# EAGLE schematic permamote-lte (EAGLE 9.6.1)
AUTHOR: NEAL JACKSON; REV: C; TITLE: PERMAMOTE

## Sheet 1 of 5: NRF
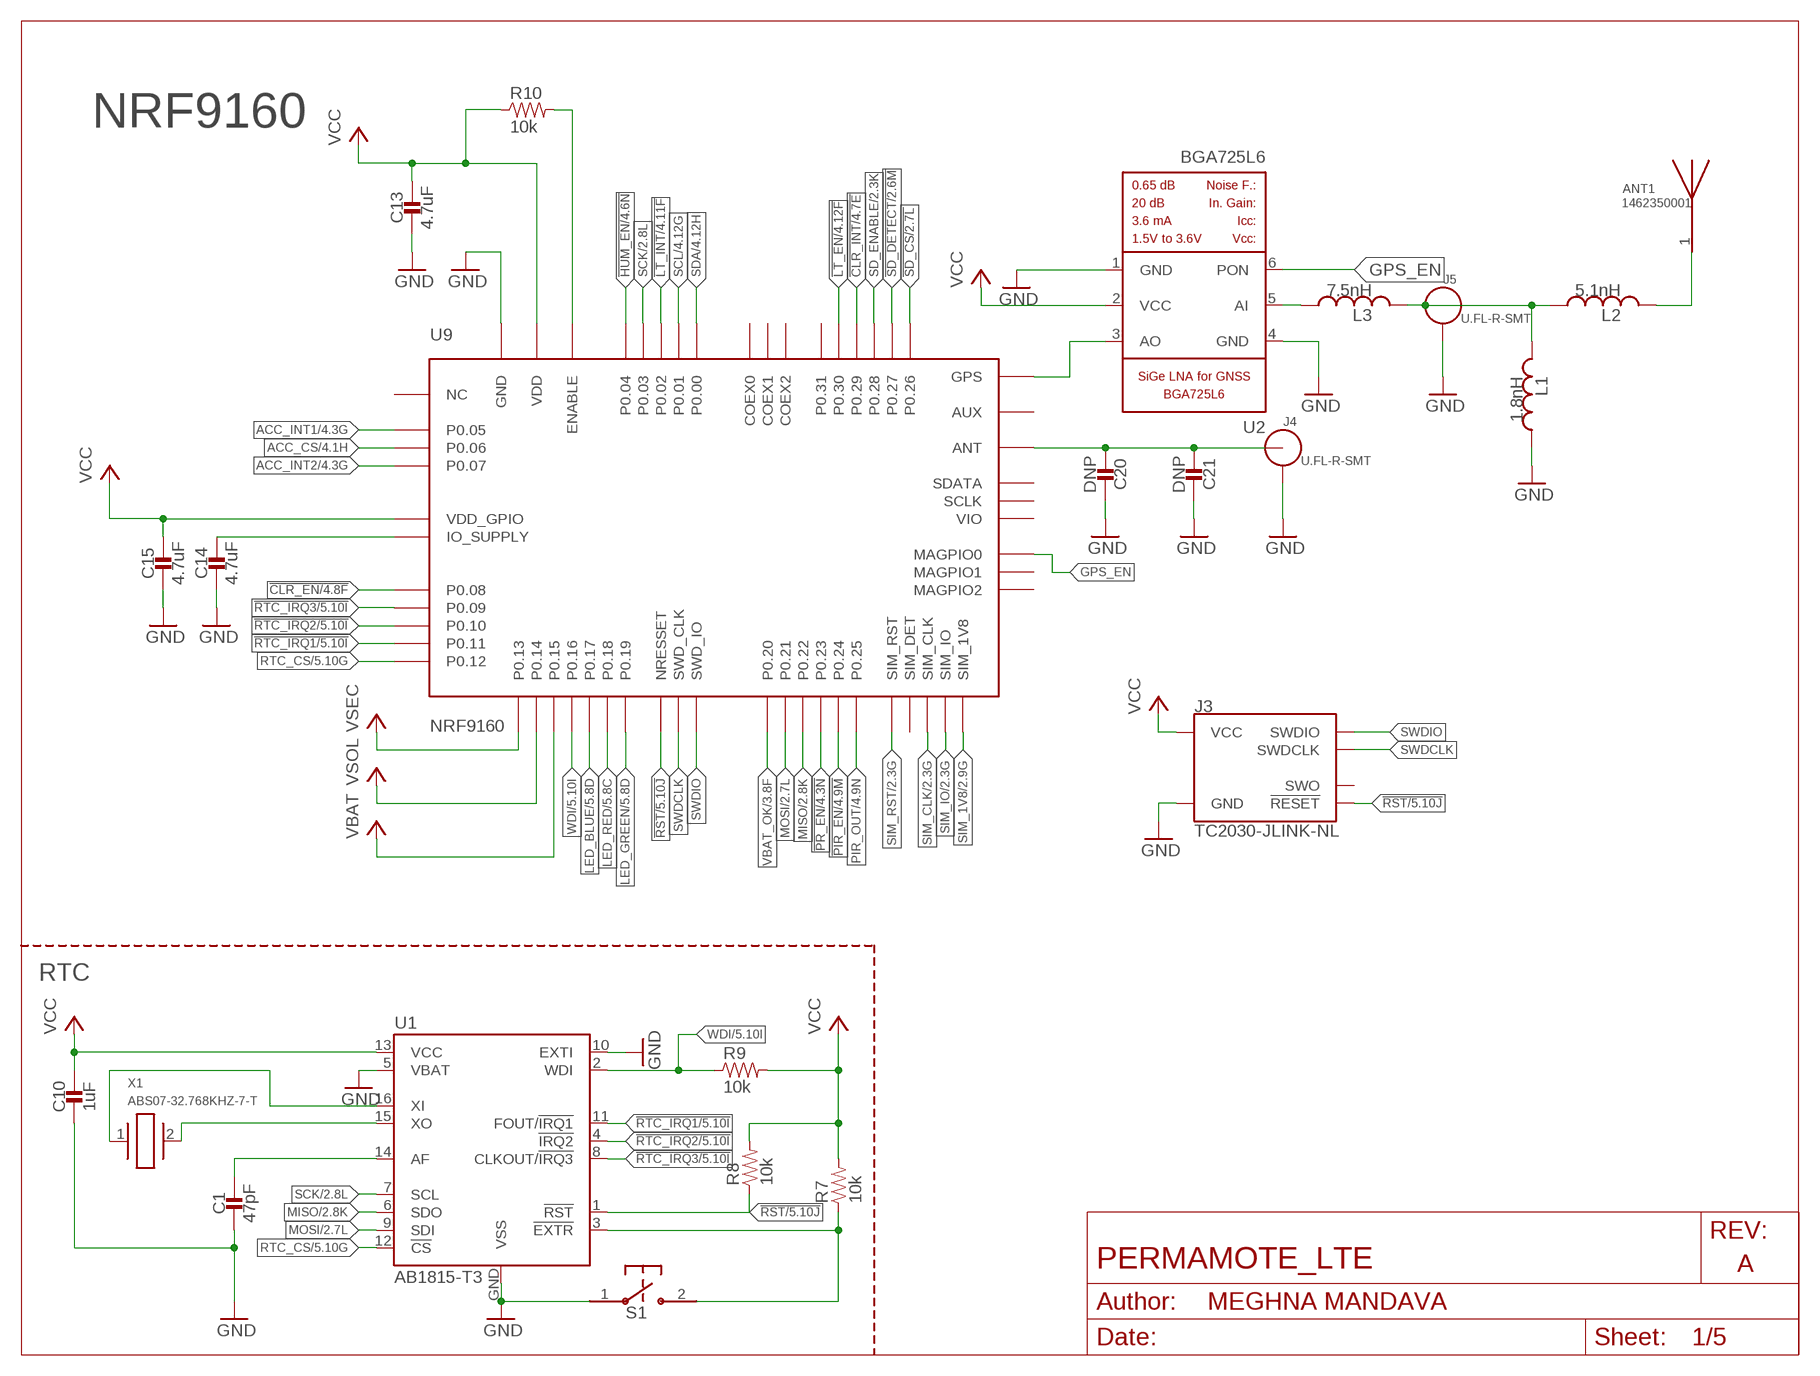
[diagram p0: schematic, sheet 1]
FRAME1 (LETTER_L_BLANK): AUTHOR: MEGHNA MANDAVA; REV: A; TITLE: PERMAMOTE_LTE

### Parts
ANT1  1462350001  [ANT_1462350001]
C1  47pF  CAPACITOR0402_CAP  [0402_CAP]
C10  1uF  CAPACITOR0402_CAP  [0402_CAP]
C13  4.7uF  CAPACITOR0402_CAP  [0402_CAP]
C14  4.7uF  CAPACITOR0402_CAP  [0402_CAP]
C15  4.7uF  CAPACITOR0402_CAP  [0402_CAP]
C20  DNP  CAPACITOR0402_CAP  [0402_CAP]
C21  DNP  CAPACITOR0402_CAP  [0402_CAP]
J3  TC2030-JLINK-NL  [TC2030-IDC-NL]
J4  U.FL-R-SMT  [U.FL_SMT]
J5  U.FL-R-SMT  [U.FL_SMT]
L1  1.8nH  INDUCTOR0402  [0402_CAP]
L2  5.1nH  INDUCTOR0402  [0402_CAP]
L3  7.5nH  INDUCTOR0402  [0402_CAP]
R7  10k  RESISTOR0402_RES  [0402_RES]
R8  10k  RESISTOR0402_RES  [0402_RES]
R9  10k  RESISTOR0402_RES  [0402_RES]
R10  10k  RESISTOR0402_RES  [0402_RES]
S1  B3U-1000P  [B3U-1000P]
U1  AB1815-T3  [QFN-16-3MM]
U2  BGA725L6  [LNA-TSLP-6-2-ORIG]
U9  NRF9160  [NRF9160]
X1  ABS07-32.768KHZ-7-T  [2-SMD]

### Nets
!CLR_EN: U9.P0.08 ; also sheet 4,5
!CLR_INT: U9.P0.29 ; also sheet 4,5
!HUM_EN: U9.P0.04 ; also sheet 4,5
!LT_EN: U9.P0.30 ; also sheet 4,5
!LT_INT: U9.P0.02 ; also sheet 4,5
!PIR_EN: U9.P0.24 ; also sheet 4,5
!PR_EN: U9.P0.23 ; also sheet 4,5
!RST: J3.3(!RESET) R8.1 U1.1(!RST) U9.NRESET(NRESSET) ; also sheet 5
!RTC_EXTR: R7.1 S1.2 U1.3(!EXTR)
!RTC_IRQ1: U1.11(FOUT/!IRQ1) U9.P0.11 ; also sheet 5
!RTC_IRQ2: U1.4(!IRQ2) U9.P0.10 ; also sheet 5
!RTC_IRQ3: U1.8(CLKOUT/!IRQ3) U9.P0.09 ; also sheet 5
!SD_CS: U9.P0.26 ; also sheet 2
!SD_DETECT: U9.P0.27 ; also sheet 2
ACC_CS: U9.P0.06 ; also sheet 4,5
ACC_INT1: U9.P0.05 ; also sheet 4,5
ACC_INT2: U9.P0.07 ; also sheet 4,5
GND: C1.2 C10.2 C13.2 C14.2 C15.2 C20.1 C21.1 J3.5(GND) J4.GND1 J4.GND2 J5.GND1 J5.GND2 L1.1 S1.1 U1.5(VBAT) U1.10(EXTI) U1.GND(VSS) U2.1(GND) U2.4(GND) U9.GND@1(GND) U9.GND@2(GND) U9.GND@3(GND) U9.GND@4(GND) U9.GND@5(GND) U9.GND@6(GND) U9.GND@7(GND) U9.GND@8(GND) U9.GND@9(GND) U9.GND@10(GND) U9.GND@11(GND) U9.GND@12(GND) U9.GND@13(GND) U9.GND@14(GND) U9.GND@15(GND) U9.GND@16(GND) U9.GND@17(GND) U9.GND@18(GND) U9.GND@19(GND) U9.GND@20(GND) U9.GND@21(GND) U9.GND@22(GND) U9.GND@23(GND) U9.GND@24(GND) U9.GND@25(GND) U9.GND@26(GND) U9.GND@27(GND) U9.GND@28(GND) U9.GND@29(GND) U9.GND@30(GND) U9.GND@31(GND) U9.GND@32(GND) U9.GND@33(GND) U9.GND@34(GND) U9.GND@35(GND) U9.GND_SHIELD@1(GND) U9.GND_SHIELD@2(GND) U9.GND_SHIELD@3(GND) U9.GND_SHIELD@4(GND) U9.GND_SHIELD@5(GND) U9.GND_SHIELD@6(GND) U9.GND_SHIELD@7(GND) U9.GND_SHIELD@8(GND) U9.GND_SHIELD@9(GND) U9.GND_SHIELD@10(GND) U9.GND_SHIELD@11(GND) U9.GND_SHIELD@12(GND) U9.GND_SHIELD@13(GND) U9.GND_SHIELD@14(GND) U9.GND_SHIELD@15(GND) U9.GND_SHIELD@16(GND) U9.GND_SHIELD@17(GND) U9.GND_SHIELD@18(GND) U9.GND_SHIELD@19(GND) U9.GND_SHIELD@20(GND) U9.GND_SHIELD@21(GND) U9.GND_SHIELD@22(GND) U9.GND_SHIELD@23(GND) U9.GND_SHIELD@24(GND) U9.GND_SHIELD@25(GND) U9.GND_SHIELD@26(GND) U9.GND_SHIELD@27(GND) U9.GND_SHIELD@28(GND) U9.GND_SHIELD@29(GND) U9.GND_SHIELD@30(GND) U9.GND_SHIELD@31(GND) U9.GND_SHIELD@32(GND) U9.GND_SHIELD@33(GND) U9.GND_SHIELD@34(GND) ; also sheet 2,3,4,5
GPS_EN: U2.6(PON) U9.MAGPIO0
LED_BLUE: U9.P0.17 ; also sheet 5
LED_GREEN: U9.P0.19 ; also sheet 5
LED_RED: U9.P0.18 ; also sheet 5
MISO: U1.6(SDO) U9.P0.22 ; also sheet 2,4,5
MOSI: U1.9(SDI) U9.P0.21 ; also sheet 2,4,5
N$1: U2.3(AO) U9.GPS
N$2: L3.1 U2.5(AI)
N$4: J5.SIG(ANT) L1.2 L2.1 L3.2
N$5: ANT1.1 L2.2
N$8: C20.2 C21.2 J4.SIG(ANT) U9.ANT
N$25: C1.1 U1.14(AF)
N$28: R10.2 U9.ENABLE
N$29: C14.1 U9.IO_SUPPLY
N$40: U1.15(XO) X1.2
N$43: U1.16(XI) X1.1
PIR_OUT: U9.P0.25 ; also sheet 4,5
RTC_CS: U1.12(!CS) U9.P0.12 ; also sheet 5
SCK: U1.7(SCL) U9.P0.03 ; also sheet 2,4,5
SCL: U9.P0.01 ; also sheet 4,5
SD_ENABLE: U9.P0.28 ; also sheet 2
SDA: U9.P0.00 ; also sheet 4,5
SIM_1V8: U9.SIM_1V8 ; also sheet 2
SIM_CLK: U9.SIM_CLK ; also sheet 2
SIM_IO: U9.SIM_IO ; also sheet 2
SIM_RST: U9.SIM_RST ; also sheet 2
SWDCLK: J3.4(SWDCLK) U9.SWDCLK(SWD_CLK)
SWDIO: J3.2(SWDIO) U9.SWDIO(SWD_IO)
VBAT: U9.P0.15 ; also sheet 3
VBAT_OK: U9.P0.20 ; also sheet 3
VCC: C10.1 C13.1 C15.1 J3.1(VCC) R7.2 R8.2 R9.2 R10.1 U1.13(VCC) U2.2(VCC) U9.VDD@1(VDD) U9.VDD@2(VDD) U9.VDD_GPIO ; also sheet 2,3,4,5
VSEC: U9.P0.13 ; also sheet 3
VSOL: U9.P0.14 ; also sheet 3,5
WDI: R9.1 U1.2(WDI) U9.P0.16 ; also sheet 5
Unconnected: J3.6(SWO) U9.AUX U9.COEX0 U9.COEX1 U9.COEX2 U9.MAGPIO1 U9.MAGPIO2 U9.NC1(NC) U9.NC2(NC) U9.NC3(NC) U9.NC4(NC) U9.NC5(NC) U9.NC6(NC) U9.NC7(NC) U9.NC8(NC) U9.NC9(NC) U9.NC10(NC) U9.NC11(NC) U9.NC12(NC) U9.NC13(NC) U9.NC14(NC) U9.NC15(NC) U9.NC16(NC) U9.NC17(NC) U9.NC18(NC) U9.NC19(NC) U9.NC20(NC) U9.NC21(NC) U9.NC22(NC) U9.NC23(NC) U9.NC24(NC) U9.NC25(NC) U9.NC26(NC) U9.NC27(NC) U9.NC28(NC) U9.NC29(NC) U9.NC30(NC) U9.NC31(NC) U9.NC32(NC) U9.NC33(NC) U9.NC34(NC) U9.NC35(NC) U9.P0.31 U9.SCLK U9.SDATA U9.SIM_DET U9.VIO

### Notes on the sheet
- NRF9160
- RTC

## Sheet 2 of 5: SIM and SD
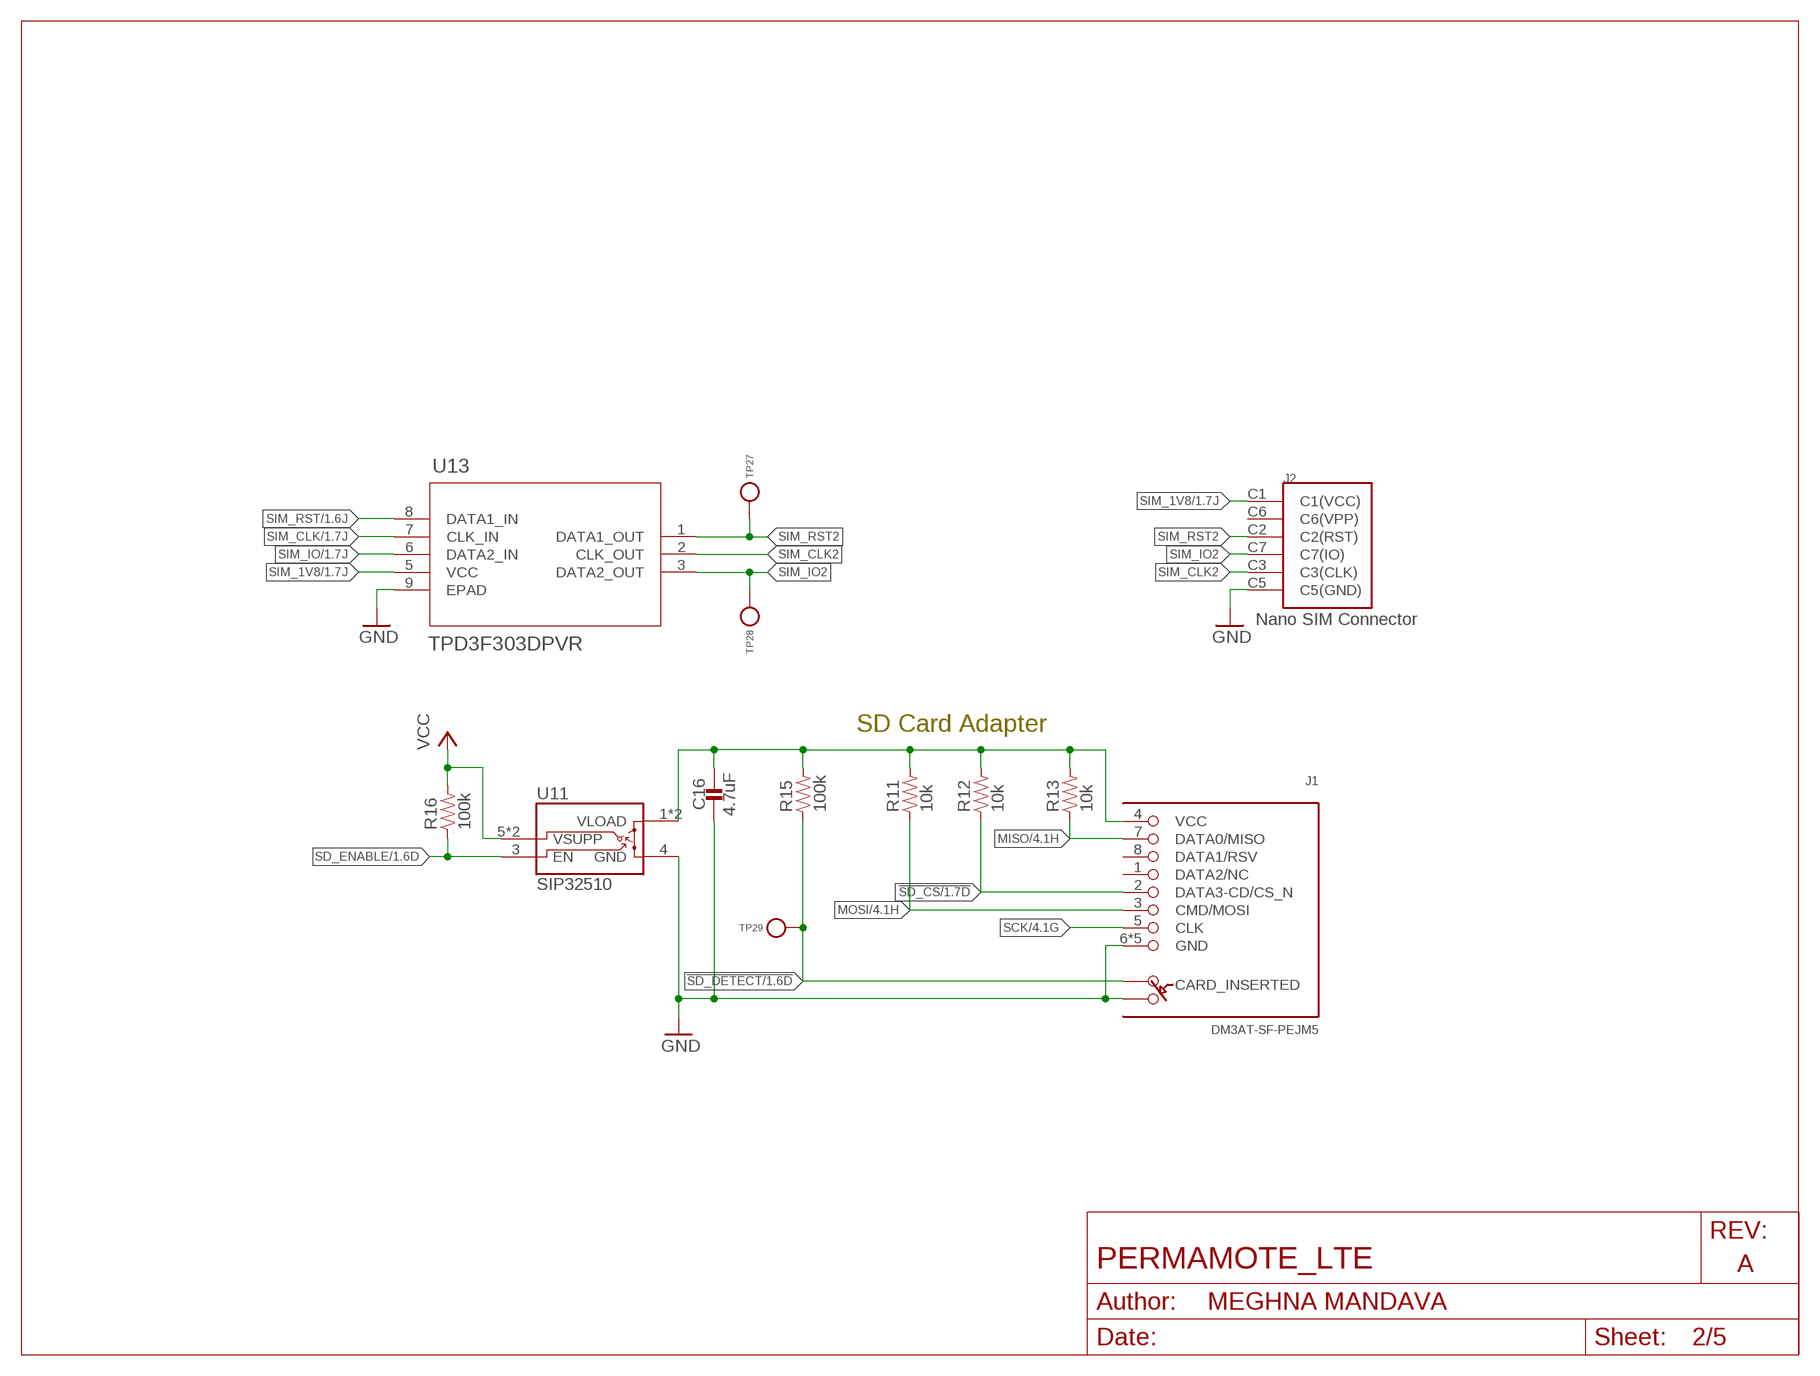
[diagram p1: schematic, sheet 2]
FRAME4 (LETTER_L_BLANK): AUTHOR: MEGHNA MANDAVA; REV: A; TITLE: PERMAMOTE_LTE

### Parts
C16  4.7uF  CAPACITOR0402_CAP  [0402_CAP]
J1  DM3AT-SF-PEJM5  [DM3AT-SF-PEJM5]
J2  NANO_SIM  [WURTH_NANO_SIM]
R11  10k  RESISTOR0402_RES  [0402_RES]
R12  10k  RESISTOR0402_RES  [0402_RES]
R13  10k  RESISTOR0402_RES  [0402_RES]
R15  100k  RESISTOR0402_RES  [0402_RES]
R16  100k  RESISTOR0402_RES  [0402_RES]
TP27  TEST-POINT  [PAD.03X.03]
TP28  TEST-POINT  [PAD.03X.03]
TP29  TEST-POINT  [PAD.03X.03]
U11  SIP32510  [TSOT23-6]
U13  TPD3F303DPVR  [DPV8_1P7X0P4]

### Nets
!SD_CS: J1.2(DATA3-CD/CS_N) R12.1 ; also sheet 1
!SD_DETECT: J1.A R15.1 TP29.P$1(TESTPOINT) ; also sheet 1
GND: C16.2 J1.6(GND) J1.B J1.MOUNT0(GND) J1.MOUNT1(GND) J1.MOUNT2(GND) J1.MOUNT3(GND) J2.C5(C5(GND)) U11.4(GND) U13.9(EPAD) ; also sheet 1,3,4,5
MISO: J1.7(DATA0/MISO) R13.1 ; also sheet 1,4,5
MOSI: J1.3(CMD/MOSI) R11.1 ; also sheet 1,4,5
N$13: C16.1 J1.4(VCC) R11.2 R12.2 R13.2 R15.2 U11.1(VLOAD) U11.2(VLOAD)
SCK: J1.5(CLK) ; also sheet 1,4,5
SD_ENABLE: R16.1 U11.3(EN) ; also sheet 1
SIM_1V8: J2.C1(C1(VCC)) U13.5(VCC) ; also sheet 1
SIM_CLK: U13.7(CLK_IN) ; also sheet 1
SIM_CLK2: J2.C3(C3(CLK)) U13.2(CLK_OUT)
SIM_IO: U13.6(DATA2_IN) ; also sheet 1
SIM_IO2: J2.C7(C7(IO)) TP28.P$1(TESTPOINT) U13.3(DATA2_OUT)
SIM_RST: U13.8(DATA1_IN) ; also sheet 1
SIM_RST2: J2.C2(C2(RST)) TP27.P$1(TESTPOINT) U13.1(DATA1_OUT)
VCC: R16.2 U11.5(VSUPP) U11.6(VSUPP) ; also sheet 1,3,4,5
Unconnected: J1.1(DATA2/NC) J1.8(DATA1/RSV) J2.C6(C6(VPP))

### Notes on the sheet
- SD Card Adapter

## Sheet 3 of 5: Power supply
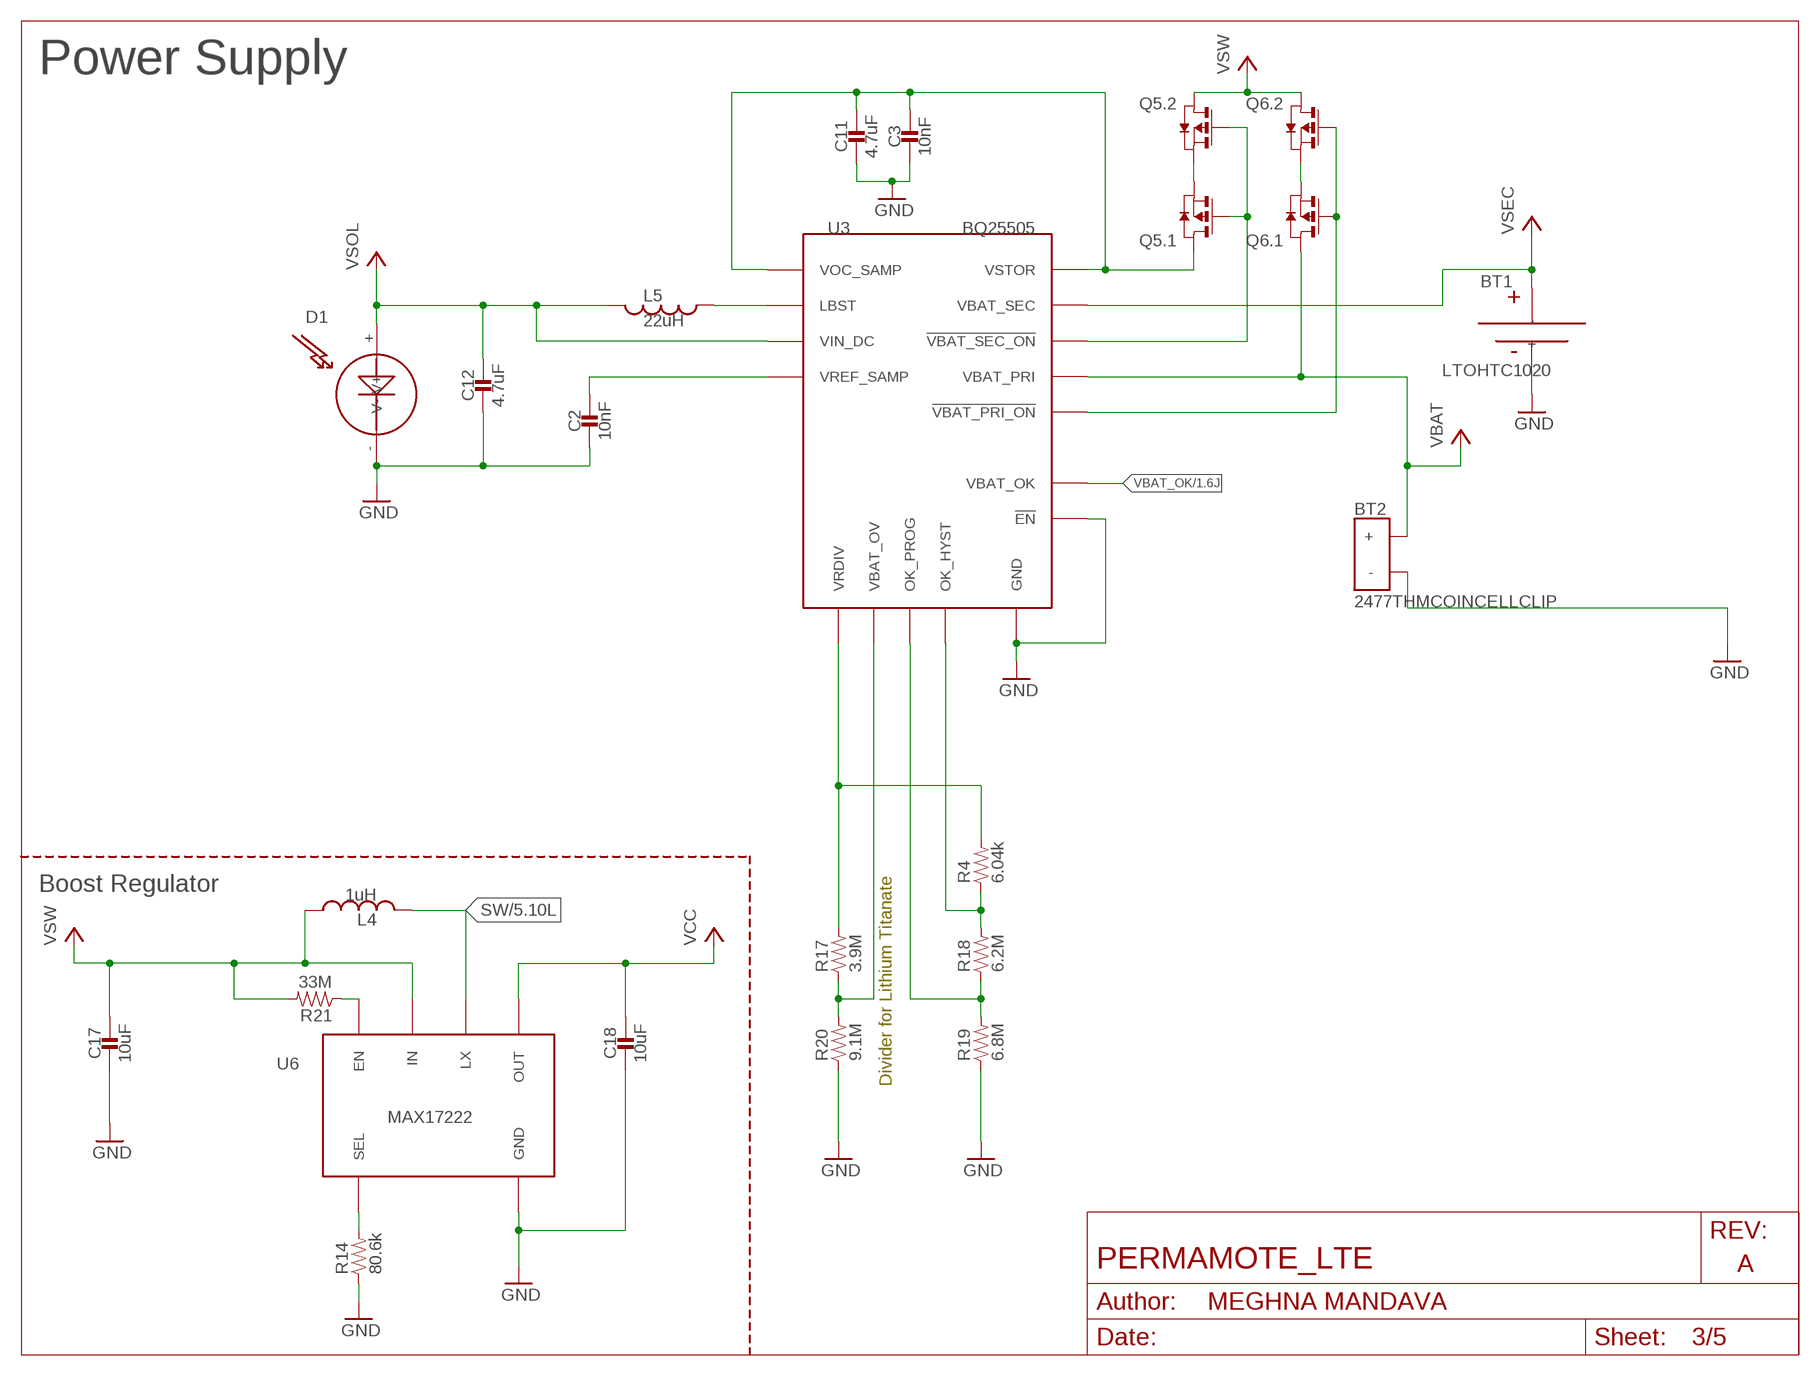
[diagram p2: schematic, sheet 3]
FRAME2 (LETTER_L_BLANK): AUTHOR: MEGHNA MANDAVA; REV: A; TITLE: PERMAMOTE_LTE

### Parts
BT1  LTOHTC1020  [1020]
BT2  2477THMCOINCELLCLIP  [2477THMCOINCLIP]
C2  10nF  CAPACITOR0402_CAP  [0402_CAP]
C3  10nF  CAPACITOR0402_CAP  [0402_CAP]
C11  4.7uF  CAPACITOR0402_CAP  [0402_CAP]
C12  4.7uF  CAPACITOR0402_CAP  [0402_CAP]
C17  10uF  CAPACITOR0603_CAP  [0603_CAP]
C18  10uF  CAPACITOR0603_CAP  [0603_CAP]
D1  SOLARCELLHOLES  [SOLAR_HOLES]
L4  1uH  INDUCTORIHL  [IHL-1212BZ-11]
L5  22uH  INDUCTOR74437324220  [74437324220]
Q5  PMDXB950UPEL  [XDFN-6]
Q6  PMDXB950UPEL  [XDFN-6]
R4  6.04k  RESISTOR0402_RES  [0402_RES]
R14  80.6k  RESISTOR0603_RES  [0603-RES]
R17  3.9M  RESISTOR0402_RES  [0402_RES]
R18  6.2M  RESISTOR0402_RES  [0402_RES]
R19  6.8M  RESISTOR0402_RES  [0402_RES]
R20  9.1M  RESISTOR0402_RES  [0402_RES]
R21  33M  RESISTOR0603_RES  [0603-RES]
U3  BQ25505  [S-PVQFN-N20-RGR]
U6  MAX17222  [UDFN-6-MAXIM]

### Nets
!VBAT_PRI_ON: Q6.2(.1:G) Q6.5(.2:G) U3.10(!VBAT_PRI_ON)
!VBAT_SEC_ON: Q5.2(.1:G) Q5.5(.2:G) U3.9(!VBAT_SEC_ON)
GND: BT1.- BT2.GND(-) C2.2 C3.2 C11.2 C12.2 C17.2 C18.2 D1.-(V-) R14.1 R19.1 R20.1 U3.1(GND) U3.5(!EN) U3.6(GND) U3.15(GND) U3.16(GND) U3.17(GND) U3.PAD(GND) U6.3(GND) ; also sheet 1,2,4,5
LBST: L5.P$1 U3.20(LBST)
N$12: R14.2 U6.4(SEL)
N$14: R21.1 U6.6(EN)
N$18: R17.1 R20.2 U3.7(VBAT_OV)
N$32: R4.2 R17.2 U3.8(VRDIV)
N$45: Q5.1(.1:S) Q5.4(.2:S)
N$53: Q6.1(.1:S) Q6.4(.2:S)
N$57: R18.1 R19.2 U3.12(OK_PROG)
N$58: R4.1 R18.2 U3.11(OK_HYST)
SW: L4.P$2 U6.2(LX) ; also sheet 5
VBAT: BT2.1(+) BT2.2(+) Q6.6(.1:D) U3.14(VBAT_PRI) ; also sheet 1
VBAT_OK: U3.13(VBAT_OK) ; also sheet 1
VCC: C18.1 U6.1(OUT) ; also sheet 1,2,4,5
VOC_SAMP_VSTOR: C3.1 C11.1 Q5.6(.1:D) U3.3(VOC_SAMP) U3.19(VSTOR)
VREF_SAMP: C2.1 U3.4(VREF_SAMP)
VSEC: BT1.+ U3.18(VBAT_SEC) ; also sheet 1
VSOL: C12.1 D1.+(V+) L5.P$2 U3.2(VIN_DC) ; also sheet 1,5
VSW: C17.1 L4.P$1 Q5.3(.2:D) Q6.3(.2:D) R21.2 U6.5(IN)

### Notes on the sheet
- Power Supply
- Boost Regulator
- Divider for Lithium Titanate

## Sheet 4 of 5: Sensors
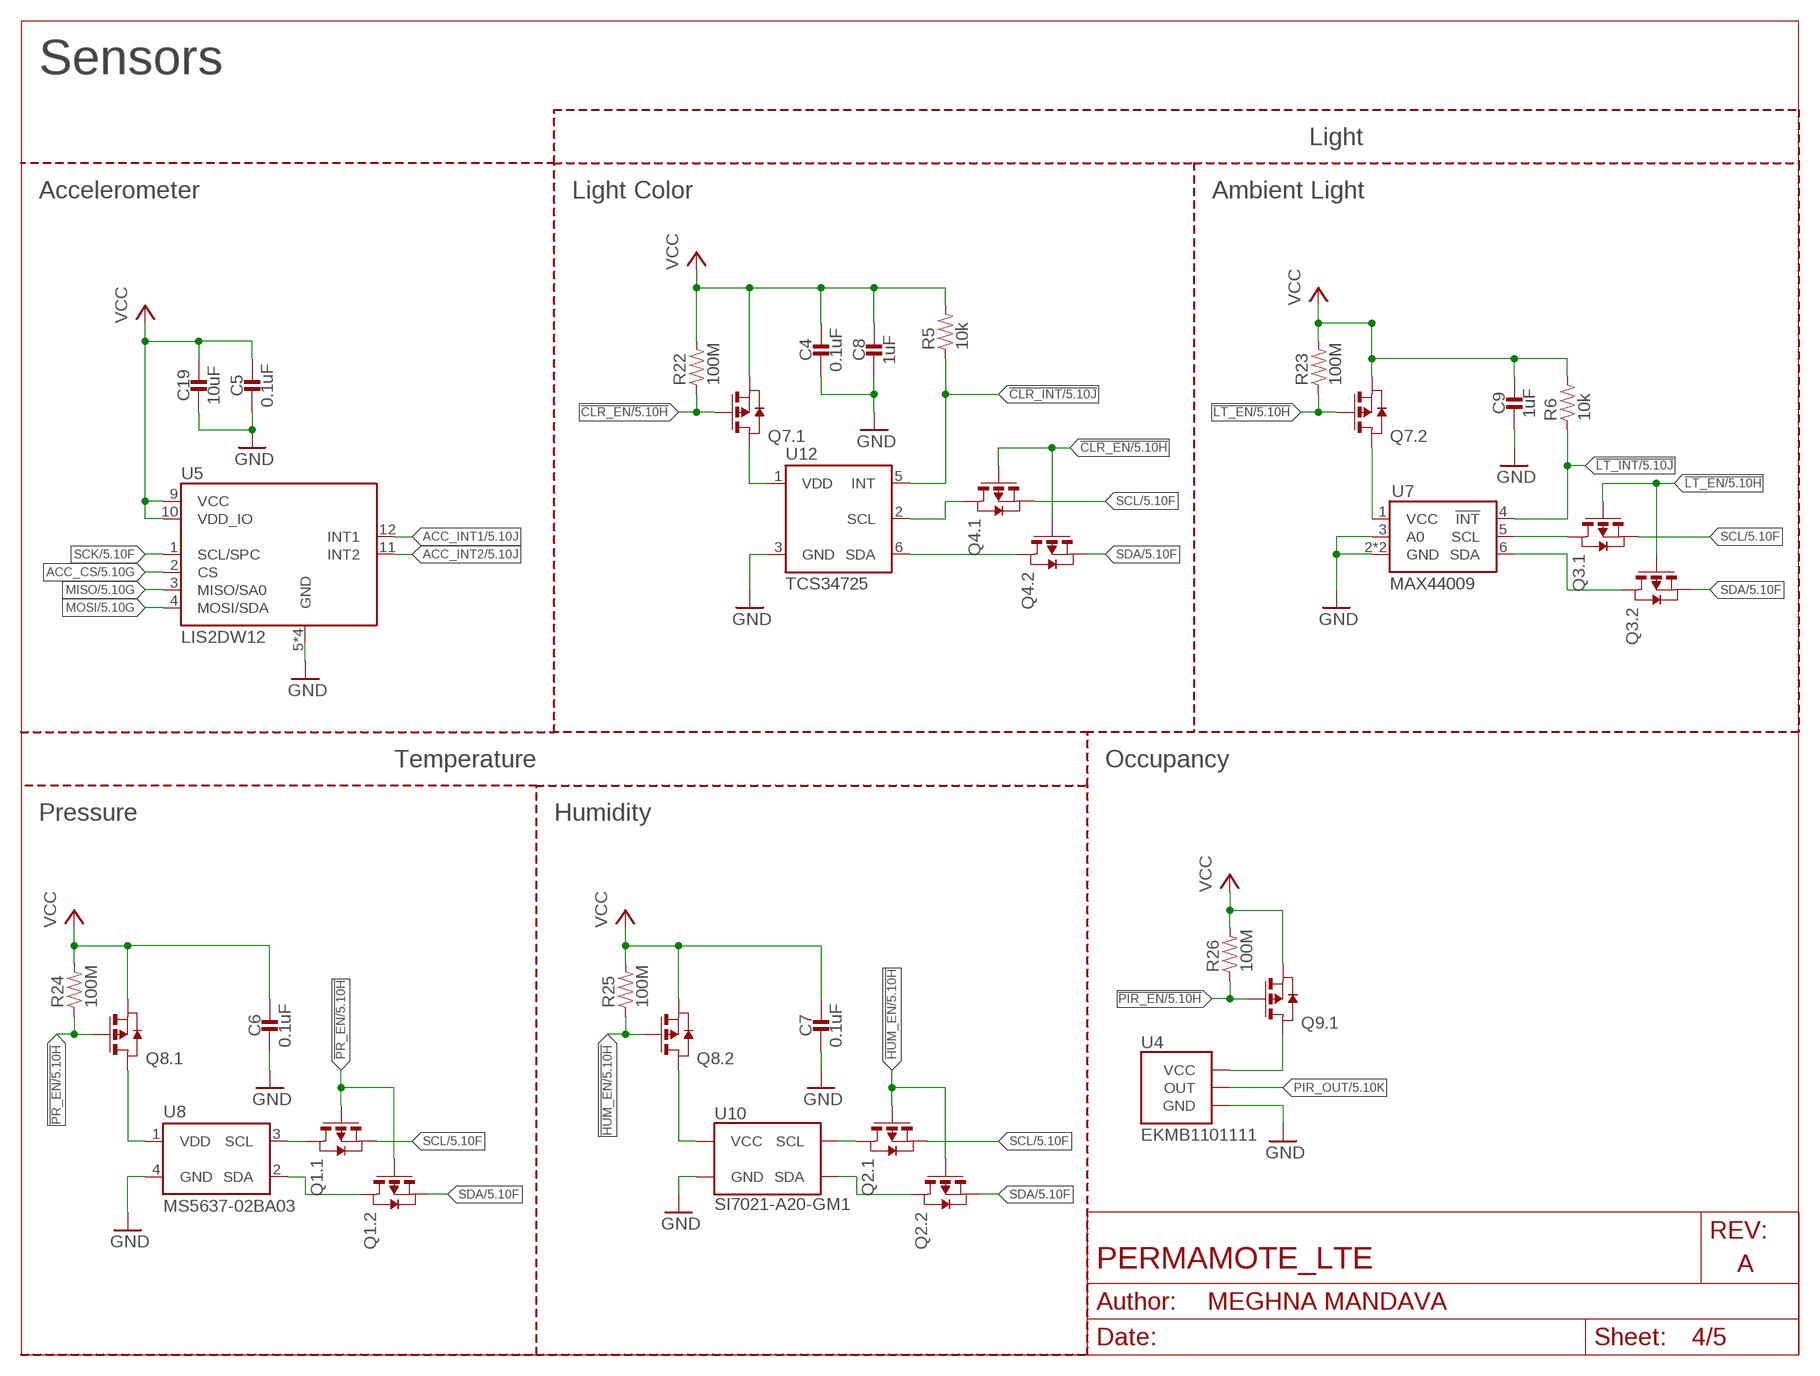
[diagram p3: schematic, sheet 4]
FRAME3 (LETTER_L_BLANK): AUTHOR: MEGHNA MANDAVA; REV: A; TITLE: PERMAMOTE_LTE

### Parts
C4  0.1uF  CAPACITOR0402_CAP  [0402_CAP]
C5  0.1uF  CAPACITOR0402_CAP  [0402_CAP]
C6  0.1uF  CAPACITOR0402_CAP  [0402_CAP]
C7  0.1uF  CAPACITOR0402_CAP  [0402_CAP]
C8  1uF  CAPACITOR0402_CAP  [0402_CAP]
C9  1uF  CAPACITOR0402_CAP  [0402_CAP]
C19  10uF  CAPACITOR0603_CAP  [0603_CAP]
Q1  PMDXB950UPEL  [XDFN-6]
Q2  PMDXB950UPEL  [XDFN-6]
Q3  PMDXB950UPEL  [XDFN-6]
Q4  PMDXB950UPEL  [XDFN-6]
Q7  PMDXB950UPEL  [XDFN-6]
Q8  PMDXB950UPEL  [XDFN-6]
Q9  PMDXB950UPEL  [XDFN-6]
R5  10k  RESISTOR0402_RES  [0402_RES]
R6  10k  RESISTOR0402_RES  [0402_RES]
R22  100M  RESISTOR0402_RES  [0402_RES]
R23  100M  RESISTOR0402_RES  [0402_RES]
R24  100M  RESISTOR0402_RES  [0402_RES]
R25  100M  RESISTOR0402_RES  [0402_RES]
R26  100M  RESISTOR0402_RES  [0402_RES]
U4  EKMB1101111  [AMN2]
U5  LIS2DW12  [LGA-12]
U7  MAX44009  [UDFN-6-EXPOSED]
U8  MS5637-02BA03  [4-SMD]
U10  SI7021-A20-GM1  [DFN-6/3MM]
U12  TCS34725  [FN-6]

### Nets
!CLR_EN: Q4.2(.1:G) Q4.5(.2:G) Q7.2(.1:G) R22.1 ; also sheet 1,5
!CLR_INT: R5.1 U12.5(INT) ; also sheet 1,5
!HUM_EN: Q2.2(.1:G) Q2.5(.2:G) Q8.5(.2:G) R25.1 ; also sheet 1,5
!LT_EN: Q3.2(.1:G) Q3.5(.2:G) Q7.5(.2:G) R23.1 ; also sheet 1,5
!LT_INT: R6.1 U7.4(!INT) ; also sheet 1,5
!PIR_EN: Q9.2(.1:G) R26.1 ; also sheet 1,5
!PR_EN: Q1.2(.1:G) Q1.5(.2:G) Q8.2(.1:G) R24.1 ; also sheet 1,5
ACC_CS: U5.2(CS) ; also sheet 1,5
ACC_INT1: U5.12(INT1) ; also sheet 1,5
ACC_INT2: U5.11(INT2) ; also sheet 1,5
GND: C4.2 C5.2 C6.2 C7.2 C8.2 C9.2 C19.2 U4.GND U5.5(GND) U5.6(GND) U5.7(GND) U5.8(GND) U7.2(GND) U7.3(A0) U7.EP(GND) U8.4(GND) U10.2(GND) U12.3(GND) ; also sheet 1,2,3,5
MISO: U5.3(MISO/SA0) ; also sheet 1,2,5
MOSI: U5.4(MOSI/SDA) ; also sheet 1,2,5
N$20: Q7.3(.2:D) U7.1(VCC)
N$21: Q8.6(.1:D) U8.1(VDD)
N$22: Q8.3(.2:D) U10.5(VCC)
N$23: Q9.6(.1:D) U4.VCC
N$31: Q7.6(.1:D) U12.1(VDD)
N$34: Q1.6(.1:D) U8.3(SCL)
N$41: Q1.3(.2:D) U8.2(SDA)
N$48: Q2.3(.2:D) U10.1(SDA)
N$50: Q2.6(.1:D) U10.6(SCL)
N$51: Q3.3(.2:D) U7.6(SDA)
N$52: Q3.6(.1:D) U7.5(SCL)
N$54: Q4.3(.2:D) U12.6(SDA)
N$55: Q4.6(.1:D) U12.2(SCL)
PIR_OUT: U4.OUT ; also sheet 1,5
SCK: U5.1(SCL/SPC) ; also sheet 1,2,5
SCL: Q1.1(.1:S) Q2.1(.1:S) Q3.1(.1:S) Q4.1(.1:S) ; also sheet 1,5
SDA: Q1.4(.2:S) Q2.4(.2:S) Q3.4(.2:S) Q4.4(.2:S) ; also sheet 1,5
VCC: C4.1 C5.1 C6.1 C7.1 C8.1 C9.1 C19.1 Q7.1(.1:S) Q7.4(.2:S) Q8.1(.1:S) Q8.4(.2:S) Q9.1(.1:S) R5.2 R6.2 R22.2 R23.2 R24.2 R25.2 R26.2 U5.9(VCC) U5.10(VDD_IO) ; also sheet 1,2,3,5
Unconnected: Q9.3(.2:D) Q9.4(.2:S) Q9.5(.2:G)

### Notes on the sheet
- Sensors
- Light
- Accelerometer | Light Color | Ambient Light
- Temperature | Occupancy
- Pressure | Humidity

## Sheet 5 of 5: Debugging
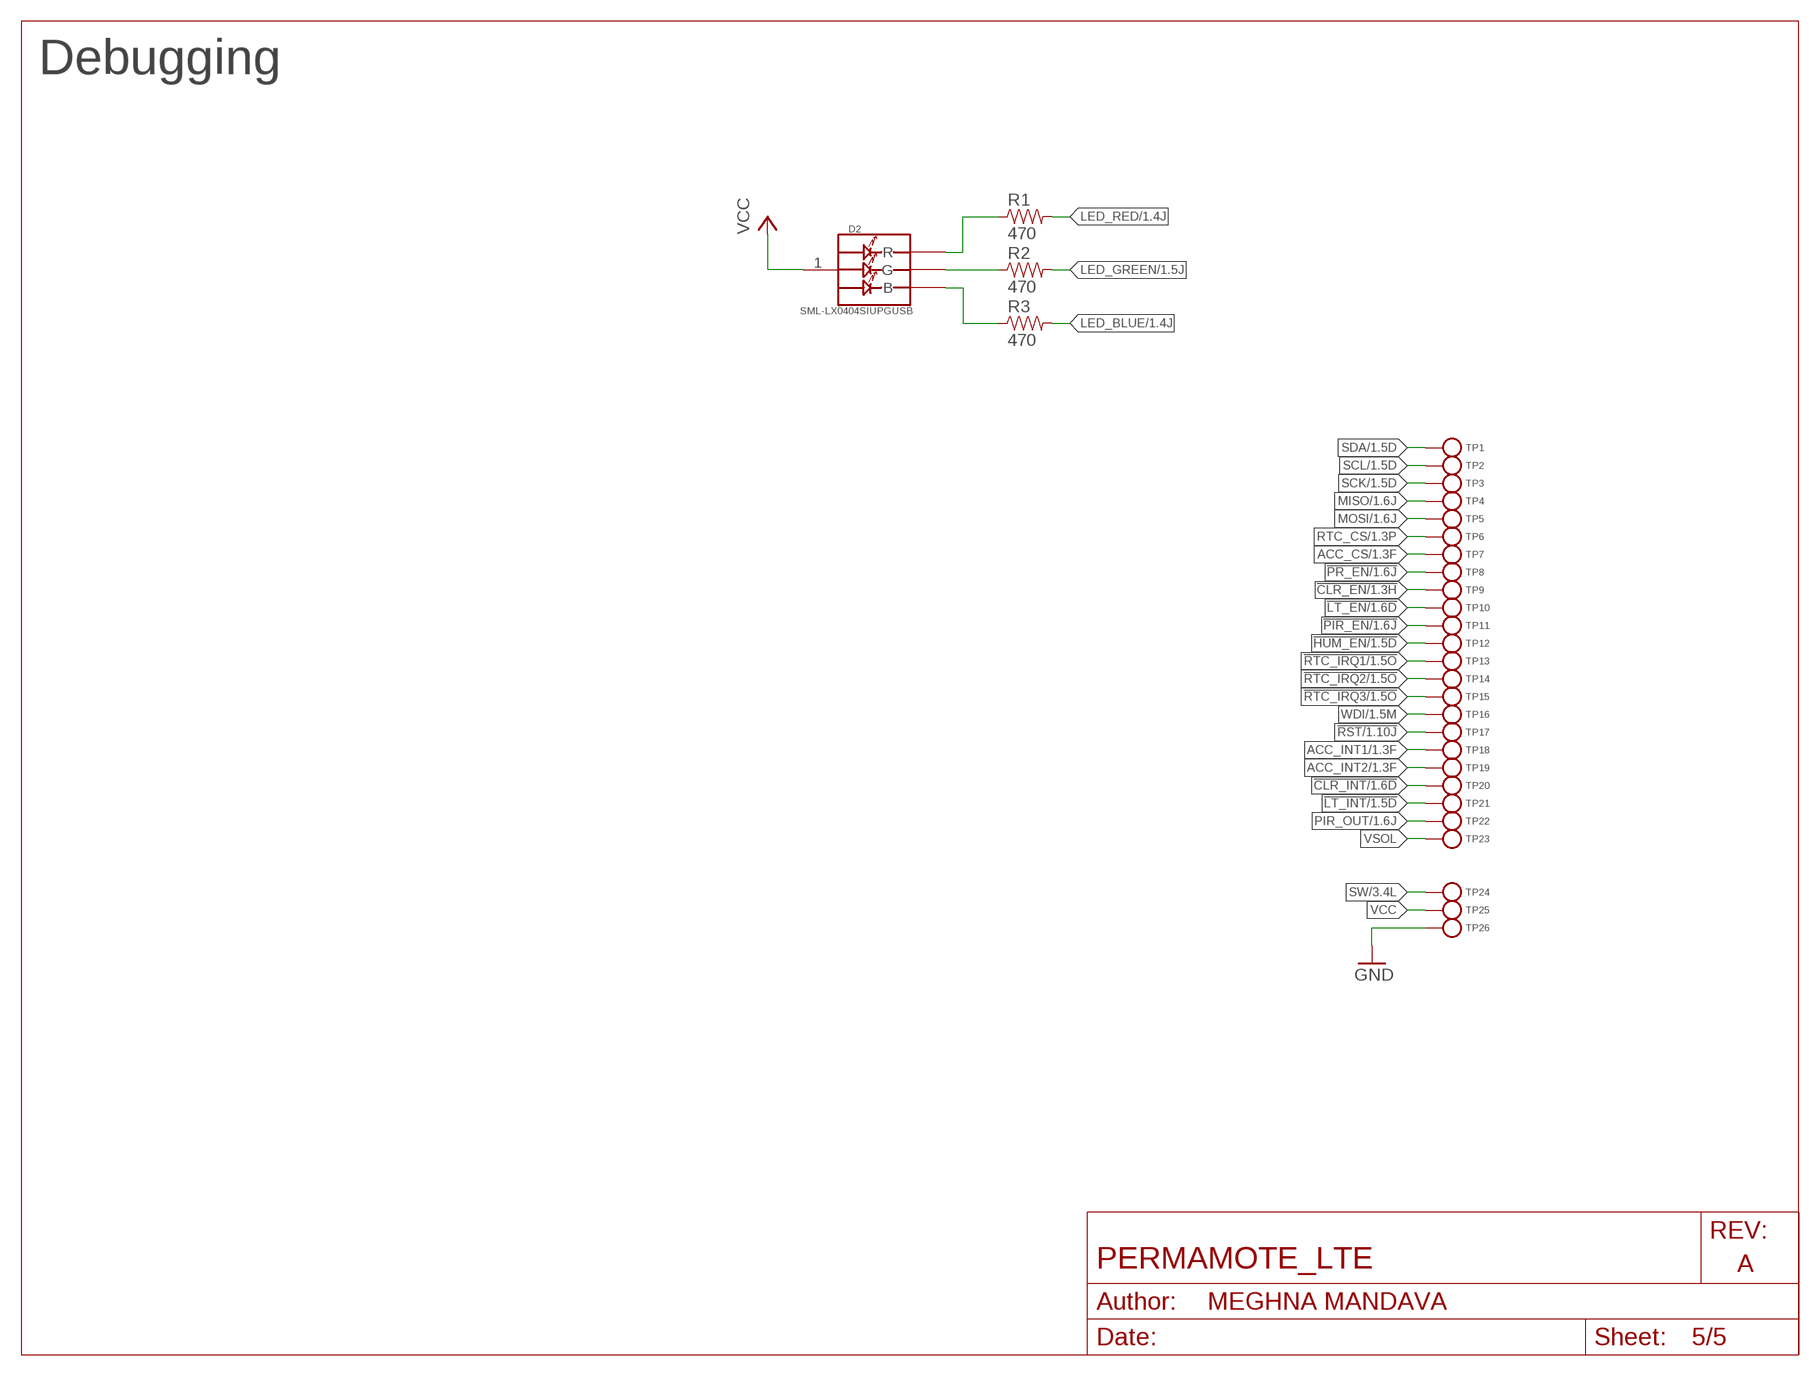
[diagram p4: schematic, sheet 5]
FRAME5 (LETTER_L_BLANK): AUTHOR: MEGHNA MANDAVA; REV: A; TITLE: PERMAMOTE_LTE

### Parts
D2  SML-LX0404SIUPGUSB  [1MM_SQ_4PAD]
R1  470  RESISTOR0402_RES  [0402_RES]
R2  470  RESISTOR0402_RES  [0402_RES]
R3  470  RESISTOR0402_RES  [0402_RES]
TP1  TEST-POINT  [PAD.03X.03]
TP2  TEST-POINT  [PAD.03X.03]
TP3  TEST-POINT  [PAD.03X.03]
TP4  TEST-POINT  [PAD.03X.03]
TP5  TEST-POINT  [PAD.03X.03]
TP6  TEST-POINT  [PAD.03X.03]
TP7  TEST-POINT  [PAD.03X.03]
TP8  TEST-POINT  [PAD.03X.03]
TP9  TEST-POINT  [PAD.03X.03]
TP10  TEST-POINT  [PAD.03X.03]
TP11  TEST-POINT  [PAD.03X.03]
TP12  TEST-POINT  [PAD.03X.03]
TP13  TEST-POINT  [PAD.03X.03]
TP14  TEST-POINT  [PAD.03X.03]
TP15  TEST-POINT  [PAD.03X.03]
TP16  TEST-POINT  [PAD.03X.03]
TP17  TEST-POINT  [PAD.03X.03]
TP18  TEST-POINT  [PAD.03X.03]
TP19  TEST-POINT  [PAD.03X.03]
TP20  TEST-POINT  [PAD.03X.03]
TP21  TEST-POINT  [PAD.03X.03]
TP22  TEST-POINT  [PAD.03X.03]
TP23  TEST-POINT  [PAD.03X.03]
TP24  TEST-POINT  [PAD.03X.03]
TP25  TEST-POINT  [PAD.03X.03]
TP26  TEST-POINT  [PAD.03X.03]

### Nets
!CLR_EN: TP9.P$1(TESTPOINT) ; also sheet 1,4
!CLR_INT: TP20.P$1(TESTPOINT) ; also sheet 1,4
!HUM_EN: TP12.P$1(TESTPOINT) ; also sheet 1,4
!LT_EN: TP10.P$1(TESTPOINT) ; also sheet 1,4
!LT_INT: TP21.P$1(TESTPOINT) ; also sheet 1,4
!PIR_EN: TP11.P$1(TESTPOINT) ; also sheet 1,4
!PR_EN: TP8.P$1(TESTPOINT) ; also sheet 1,4
!RST: TP17.P$1(TESTPOINT) ; also sheet 1
!RTC_IRQ1: TP13.P$1(TESTPOINT) ; also sheet 1
!RTC_IRQ2: TP14.P$1(TESTPOINT) ; also sheet 1
!RTC_IRQ3: TP15.P$1(TESTPOINT) ; also sheet 1
ACC_CS: TP7.P$1(TESTPOINT) ; also sheet 1,4
ACC_INT1: TP18.P$1(TESTPOINT) ; also sheet 1,4
ACC_INT2: TP19.P$1(TESTPOINT) ; also sheet 1,4
GND: TP26.P$1(TESTPOINT) ; also sheet 1,2,3,4
LED_BLUE: R3.2 ; also sheet 1
LED_GREEN: R2.2 ; also sheet 1
LED_RED: R1.2 ; also sheet 1
MISO: TP4.P$1(TESTPOINT) ; also sheet 1,2,4
MOSI: TP5.P$1(TESTPOINT) ; also sheet 1,2,4
N$15: D2.2(R) R1.1
N$17: D2.4(G) R2.1
N$19: D2.3(B) R3.1
PIR_OUT: TP22.P$1(TESTPOINT) ; also sheet 1,4
RTC_CS: TP6.P$1(TESTPOINT) ; also sheet 1
SCK: TP3.P$1(TESTPOINT) ; also sheet 1,2,4
SCL: TP2.P$1(TESTPOINT) ; also sheet 1,4
SDA: TP1.P$1(TESTPOINT) ; also sheet 1,4
SW: TP24.P$1(TESTPOINT) ; also sheet 3
VCC: D2.1(VDD) TP25.P$1(TESTPOINT) ; also sheet 1,2,3,4
VSOL: TP23.P$1(TESTPOINT) ; also sheet 1,3
WDI: TP16.P$1(TESTPOINT) ; also sheet 1

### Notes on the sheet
- Debugging

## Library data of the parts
ANT1 = chips:1462350001: Antenna GPS 1.4dBi Gain 1578MHz SMD T/R; DESCRIPTION: Antenna GPS 1.4dBi Gain 1578MHz SMD T/R; DIGI-KEY_PART_NUMBER: WM15009CT-ND; DIGI-KEY_PURCHASE_URL: https://www.digikey.com/product-detail/en/molex/1462350001/WM15009CT-ND/6159255?utm_source=snapeda&utm_medium=aggregator&utm_campaign=symbol; DIGIKEY: WM15009CT-ND; MF: Molex; MP: 1462350001; MPN: 1462350001; PACKAGE: None
BT1 = batteries:LTOHTC
BT2 = batteries:2477THMCOINCELLCLIP: Battery clip for 2477 Coin Cell; DIGIKEY: 36-3039-ND; MANUFACTURER: Keystone; MPN: 3039
C1 = passives:CAPACITOR: SMD Capacitor; DIGIKEY: 490-5942-1-ND; MPN: GRM1555C1H470JA01D
C2 C3 = passives:CAPACITOR: SMD Capacitor; DIGIKEY: 490-4516-1-ND; MPN: GRM155R71H103KA88D
C4-C7 = passives:CAPACITOR: SMD Capacitor; DIGIKEY: 490-6328-1-ND; MPN: GRM155R71C104KA88J
C8-C10 = passives:CAPACITOR: SMD Capacitor; DIGIKEY: 490-7195-1-ND; MPN: GRM155R70G105KA12D
C11-C16 = passives:CAPACITOR: SMD Capacitor; DIGIKEY: 445-5947-1-ND; MPN: C1005X5R0J475K050BC
C17-C19 = passives:CAPACITOR: SMD Capacitor; DIGIKEY: 490-3896-1-ND; MPN: GRM188R60J106ME47D
C20 C21 = passives:CAPACITOR: SMD Capacitor
D1 = permamote:SOLARCELL: Generic solar cell; DIGIKEY: 869-1001-ND; MPN: AM-1454CA
D2 = leds:SML-LX0404SIUPGUSB: 1mm^2 RGB LED; DIGIKEY: 67-2125-1-ND; MANUFACTURER: Lumex Opto; MPN: SML-LX0404SIUPGUSB
J1 = connector:DM3AT-SF-PEJM5: CONN MICRO SD R/A PUSH-PUSH SMD; DESCRIPTION: CONN MICRO SD CARD PUSH-PUSH R/A; DIGIKEY: HR1964CT-ND; MANUFACTURER: Hirose Electric Co Ltd; MPN: DM3AT-SF-PEJM5
J2 = signpost:NANO_SIM: WURTH Nano SIM Connector; DIGIKEY: 732-5954-1-ND; MANUFACTURER: Wurth; MPN: 693043020611
J3 = connector:TC2030-JLINK
J4 J5 = connector:U.FL-R-SMT: U.FL-R-SMT Antenna Connector; DIGIKEY: H122041-ND; MANUFACTURER: Hirose; MPN: U.FL-R-SMT-1(01)
L1 = passives:INDUCTOR: A very specific inductor; DIGIKEY: 490-2613-1-ND; MPN: LQG15HS1N8S02D
L2 = passives:INDUCTOR: A very specific inductor; DIGIKEY: 490-6564-1-ND; MPN: LQG15HN5N1S02D
L3 = passives:INDUCTOR: A very specific inductor; DIGIKEY: 490-6565-1-ND; MPN: LQG15HN7N5J02D
L4 = passives:INDUCTOR: A very specific inductor; DIGIKEY: 541-1319-1-ND; MANUFACTURER: Vishay Dale; MPN: IHLP1212BZER1R0M11
L5 = passives:INDUCTOR: A very specific inductor; DIGIKEY: 732-3340-1-ND; MPN: 74437324220
Q1-Q9 = fets:PMDXB950UPEL: 20 V 500mA, dual P-channel Trench MOSFET; DIGIKEY: 1727-2601-1-ND; MANUFACTURER: NEXPERIA; MPN: PMDXB950UPELZ
R1-R3 = passives:RESISTOR: Resistor; DIGIKEY: 311-470JRCT-ND; MPN: RC0402JR-07470RL
R4 = passives:RESISTOR: Resistor; DIGIKEY: YAG2293CT-ND; MPN: RC0402FR-076K04L
R5-R13 = passives:RESISTOR: Resistor; DIGIKEY: 311-10KJRCT-ND; MPN: RC0402JR-0710KL
R14 = passives:RESISTOR: Resistor; DIGIKEY: 311-80.6KHRCT-ND; MPN: RC0603FR-0780K6L
R15 R16 = passives:RESISTOR: Resistor; DESCRIPTION: RES SMD 100K OHM 1% 1/5W 0402; DIGIKEY: 541-100KYCT-ND; MANUFACTURER: Vishay Dale; MPN: CRCW0402100KFKEDHP
R17 = passives:RESISTOR: Resistor; DIGIKEY: YAG3301CT-ND; MPN: RC0402JR-073M9L
R18 = passives:RESISTOR: Resistor; DIGIKEY: YAG3309CT-ND; MPN: RC0402JR-076M2L
R19 = passives:RESISTOR: Resistor; DIGIKEY: YAG3310CT-ND; MPN: RC0402JR-076M8L
R20 = passives:RESISTOR: Resistor; DIGIKEY: YAG3322CT-ND; MPN: RC0402JR-079M1L
R21 = passives:RESISTOR: Resistor; DIGIKEY: HMC0603JT33M0CT-ND; MPN: HMC0603JT33M0
R22-R26 = passives:RESISTOR: Resistor; DIGIKEY: 541-100MAHCT-ND; MPN: HMC0402JT100M
S1 = switches:B3U: Switch; DIGIKEY: SW1020CT-ND; MANUFACTURER: Omron; MPN: B3U-1000P
TP1-TP29 = headers:TEST-POINT
U1 = chips:AB1815-T3: Ultra-low current RTC. 55nA quiescent @ 3V. 1.5-3.6V input.; DIGIKEY: 535-11936-1-ND; MANUFACTURER: Abracon; MPN: AB1815-T3
U2 = chips:BGA725L6; DIGIKEY: BGA725L6E6327FTSA1CT-ND; MANUFACTURER: Infineon Technologies; MPN: BGA725L6E6327FTSA1
U3 = chips:BQ25505: EH front end for switching between primary and secondary cells; DIGIKEY: 296-37078-1-ND; MANUFACTURER: TI; MPN: BQ25505RGRR
U4 = chips:EKMB: Passive infrared human detection sensor with built-in amp.; DIGIKEY: 255-3065-ND; MANUFACTURER: PANASONIC; MPN: EKMB1101111
U5 = chips:LIS2DW12: ultra low power 3 axis accelerometer; DIGIKEY: 497-17718-6-ND; MANUFACTURER: STMicroelectronics; MOUSER: 511-LIS2DW12TR; MPN: LIS2DW12TR
U6 = chips:MAX17222: Very high efficiency, very low power boost converter suitable for EH applications; DIGIKEY: MAX17222ELT+TCT-ND; MANUFACTURER: MAXIM INTEGRATED; MPN: MAX17222ELT+T
U7 = chips:MAX44009: low power ambient light sensor; DIGIKEY: MAX44009EDT+TCT-ND; MANUFACTURER: MAXIM; MPN: MAX44009EDT+T
U8 = chips:MS5637-02BA03: low power pressure sensor; DIGIKEY: 223-1199-1-ND; MANUFACTURER: TE CONNECTIVITY; MPN: MS563702BA03-50
U9 = chips:NRF9160; DIGIKEY: 1490-1076-1-ND; MANUFACTURER: Nordic Semiconductor; MPN: NRF9160-SICA-R7
U10 = chips:SI7021: IC TEMP SENSOR RH 2% DFN; DIGIKEY: 336-3141-ND; MOUSER: 634-SI7021-A20-GM1; MPN: SI7021-A20-GM1
U11 = chips:SIP32510: Load switch, slew rate controlled. By Vishay; DESCRIPTION: IC LOAD SWITCH SOT23-6; DIGIKEY: SIP32510DT-T1-GE3CT-ND; MANUFACTURER: Vishay; MPN: SIP32510DT-T1-GE3
U12 = chips:TCS34725: Color Light-to-Digital Converter with IR Filter; DIGIKEY: TCS34725FNCT-ND; MPN: TCS34725FN
U13 = chips:TPD3F303DPVR; DIGIKEY: 296-28299-1-ND; MANUFACTURER_PART_NUMBER: TPD3F303DPVR; MPN: TPD3F303DPVR; VENDOR: Texas Instruments
X1 = crystals:ABS07-32.768KHZ: 32.768kHz Crystal; DIGIKEY: 535-9543-1-ND; MANUFACTURER: ABRACON; MPN: ABS07-32.768KHZ-7-T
